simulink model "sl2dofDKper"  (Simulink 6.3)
settings: Solver=ode3  SolverMode=SingleTasking  StartTime=0.0  StopTime=dkt2  RelTol=1e-2  AbsTol=1e-3
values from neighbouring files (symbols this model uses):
  b_kdk1fw = [b_kdk1(degb_kdk1)]    [Getkdkdp.m]
  dkdst2 = 120    [runme.m]    (also in dkdata.m = 0)
  dkdsv2 = 0.2    [runme.m]    (also in dkdata.m = 0)
  dkrst2 = 1    [runme.m]    (also in dkdata.m = 0)
  dkrsv2 = 1    [runme.m]    (also in dkdata.m = 0)
  dkt2 = 200    [runme.m]    (also in dkdata.m = 0)
  m0dk = 1    [runme.m]    (also in dkccpe.m = 0)
  m1dk = 0    [runme.m]    (also in dkccpe.m)
  m2dk = 0    [runme.m]    (also in dkccpe.m)
  m3dk = 0    [runme.m]    (also in dkccpe.m)
  r0dk = 1    [runme.m]    (also in dkccpe.m = 0)
  r1dk = 0    [runme.m]    (also in dkccpe.m)
  r2dk = 0    [runme.m]    (also in dkccpe.m)
  r3dk = 0    [runme.m]    (also in dkccpe.m)
  Td = Tdtmp    (= 0)    [gsdata.m]    (also in runme.m = 4)
undefined symbols (not defined in the file or in its folder): a_kdk1, a_kdk2, b_kdk1, b_kdk2

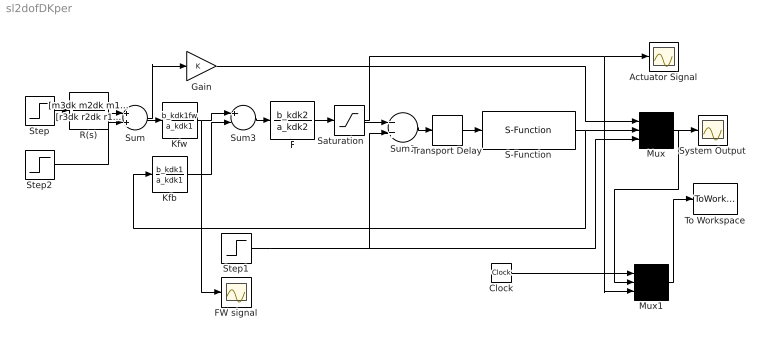
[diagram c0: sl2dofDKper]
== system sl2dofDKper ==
  Actuator Signal : Scope
  Clock : Clock
  F : TransferFcn  Numerator=b_kdk2  Denominator=a_kdk2
  FW signal : Scope
  Gain : Gain
  Kfb : TransferFcn  Numerator=b_kdk1  Denominator=a_kdk1
  Kfw : TransferFcn  Numerator=b_kdk1fw  Denominator=a_kdk1
  Mux : Mux  Inputs=3
  Mux1 : Mux  Inputs=3
  R(s) : TransferFcn  Numerator=[m3dk m2dk m1dk m0dk]  Denominator=[r3dk r2dk r1dk r0dk]
  S-Function : S-Function  FunctionName=sfperiodic
  Saturation : Saturate  UpperLimit=10  LowerLimit=-10
  Step : Step  Time=dkrst2  After=dkrsv2  SampleTime=0
  Step1 : Step  Time=400  After=0  SampleTime=0
  Step2 : Step  Time=dkdst2  After=dkdsv2  SampleTime=0
  Sum : Sum
  Sum1 : Sum
  Sum3 : Sum  Inputs=+-
  System Output : Scope
  To Workspace : ToWorkspace  VariableName=o4  SampleTime=dkt2/10000  SaveFormat=Array
  Transport Delay : TransportDelay  DelayTime=Td  BufferSize=5000
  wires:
  Gain/1 -> Mux/1
  Sum1/1 -> Transport Delay/1
  Step1/1 -> Sum1/2, Mux/3
  Mux/1 -> System Output/1, Mux1/2
  Mux1/1 -> To Workspace/1
  Clock/1 -> Mux1/1
  Transport Delay/1 -> S-Function/1
  S-Function/1 -> Mux/2, Kfb/1
  Kfw/1 -> Sum3/1, FW signal/1
  Sum/1 -> Kfw/1, Gain/1
  Kfb/1 -> Sum3/2
  Saturation/1 -> Sum1/1, Actuator Signal/1, Mux1/3
  Sum3/1 -> F/1
  F/1 -> Saturation/1
  R(s)/1 -> Sum/1
  Step/1 -> R(s)/1
  Step2/1 -> Sum/2
